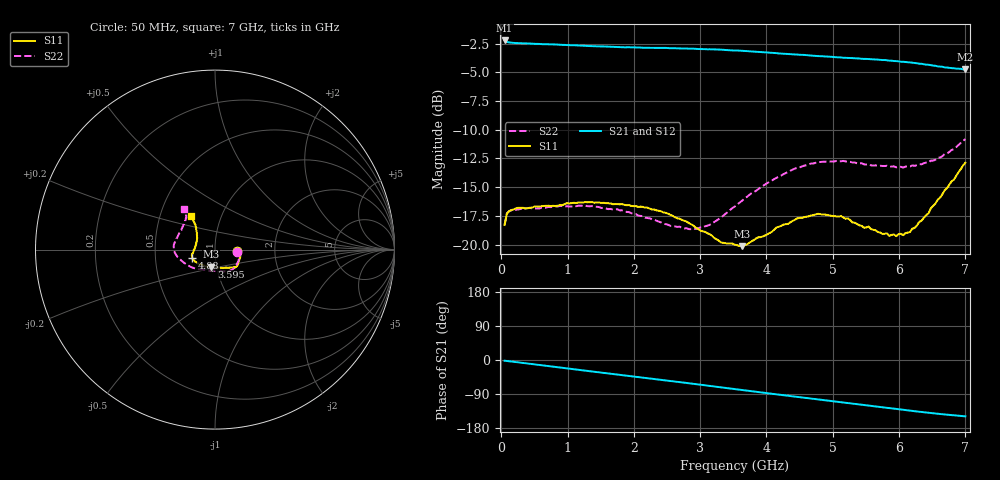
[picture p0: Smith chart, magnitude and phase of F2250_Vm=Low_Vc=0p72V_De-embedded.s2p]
! Integrated Device Technology
! Corporate Headquarters
! 6024 Silver Creek Valley Road
! San Jose, CA 95138  USA
! Phone:  1-408-284-8200
! Toll Free:  1-800-223-1366
! Webpage:  http://www.idt.com/
! Timing and RF Division
! 515 Groton Road, Suite 102
! Westford, MA 01886-6024
! Device:  F2250
! Description: Voltage Variable RF Attenuator
! Frequency:  50.0 -  6000.00 MHz
! Package:  3x3 mm Thin QFN Plastic Package: 16 pin
! Ports:  2 RF, 3 DC
!  Pin  1  = GND
!  Pin  2  = NC
!  Pin  3  = RF1  = Port 1
!  Pin  4  = NC
!  Pin  5  = GND
!  Pin  6  = GND
!  Pin  7  = GND
!  Pin  8  = GND
!  Pin  9  = NC
!  Pin 10  = RF2  = Port 2
!  Pin 11  = NC
!  Pin 12  = GND
!  Pin 13  = GND
!  Pin 14  = VCNTRL
!  Pin 15  = VDD
!  Pin 16  = VMODE
! Vcntrl:  0.720 Volts
! Vmode:  +0.000 Volts
! Vdd:  +3.30  Volts
! Current:  1.152 mA
! Data:  The device was measured on a the F2250 evaluation board which has
!  individual transmission lines to the RF pins.  Data was collected
!  using a calibrated network analyzer.  The evaluation board was
!  de-embedded using a TRL calibration technique.
!  The reference plane is the edge of the package pin.
! Misc:  SN 10
!  Action Tracker AT0258
! Date Measured:  2014-11-26
! Date:  2015-10-15  MJV
! Note:
!  Integrated Device Technology supplies this data as a sample of measured
!  data at the package pin for this product.  Your particular data for this
!  product may vary.
!  Data was taken at 25 degrees C.
!  Integrated Device Technology reserves the right to change this data at anytime.
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# GHz S dB R 50
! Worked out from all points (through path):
!   201 points, 50 MHz to 7 GHz, reference 50 ohm
!   highest |S21| = -2.23 dB at 50 MHz (marker M1); lowest = -4.8 dB at 7 GHz (marker M2)
!   group delay of S21, straight-line fit = 59.7 ps
!   lowest |S11| = -20.1 dB at 3.629 GHz (marker M3), VSWR 1.22, Z = 46.9 - j9.07 ohm
!   |S11| at or under -10 dB: start of sweep to end of sweep
!   |S22| runs from -18.7 to -10.8 dB; largest |S21 - S12| = 0.0019
!   S11 on the Smith chart (normalised r, x): 50 MHz: 1.28, -0.02; 3.595 GHz: 0.95, -0.19; 4.88 GHz: 0.77, -0.07; 7 GHz: 0.72, +0.28
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0.05  -18.29 -4.1  -2.23 -1.9  -2.24 -1.9  -18.27 -5.5
0.08475  -17.30 -4.3  -2.36 -2.6  -2.36 -2.5  -17.28 -5.3
0.22375  -16.83 -7.9  -2.46 -5.5  -2.45 -5.5  -16.96 -10.2
0.77975  -16.63 -24.0  -2.58 -17.7  -2.57 -17.7  -16.73 -31.4
1.2315  -16.34 -34.9  -2.69 -27.4  -2.69 -27.4  -16.63 -47.1
1.75275  -16.48 -41.4  -2.81 -38.4  -2.80 -38.4  -16.93 -58.8
2.37825  -17.06 -45.4  -2.88 -51.5  -2.88 -51.5  -18.01 -72.3
2.83  -18.14 -54.4  -2.95 -61.4  -2.95 -61.4  -18.66 -91.6
3.0385  -18.85 -63.3  -2.99 -66.0  -2.98 -66.0  -18.52 -104.1
3.3165  -19.83 -79.9  -3.03 -72.2  -3.04 -72.2  -17.64 -121.3
3.525  -20.01 -94.9  -3.11 -76.8  -3.11 -76.8  -16.68 -133.1
3.5945  -20.13 -100.5  -3.12 -78.4  -3.13 -78.4  -16.35 -136.5
3.62925  -20.14 -103.3  -3.13 -79.2  -3.14 -79.2  -16.20 -138.0
4.1505  -18.51 -136.7  -3.34 -90.6  -3.34 -90.6  -14.19 -161.0
4.7065  -17.43 -156.7  -3.56 -102.6  -3.57 -102.6  -12.94 -176.5
4.88025  -17.39 -160.9  -3.63 -106.3  -3.63 -106.3  -12.78 179.5
5.1235  -17.52 -166.6  -3.71 -111.5  -3.72 -111.5  -12.75 174.0
5.85325  -19.24 168.7  -3.99 -126.9  -3.99 -126.9  -13.23 156.3
6.06175  -19.18 157.9  -4.09 -131.3  -4.09 -131.4  -13.30 150.0
6.2355  -18.56 146.6  -4.19 -135.0  -4.21 -135.1  -13.14 144.1
6.61775  -15.92 130.7  -4.50 -142.5  -4.51 -142.5  -12.43 131.9
7  -12.87 125.6  -4.75 -148.7  -4.75 -148.7  -10.82 127.5
